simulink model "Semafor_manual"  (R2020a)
settings: Solver=VariableStepAuto  StartTime=0.0  StopTime=inf  RelTol=1e-3

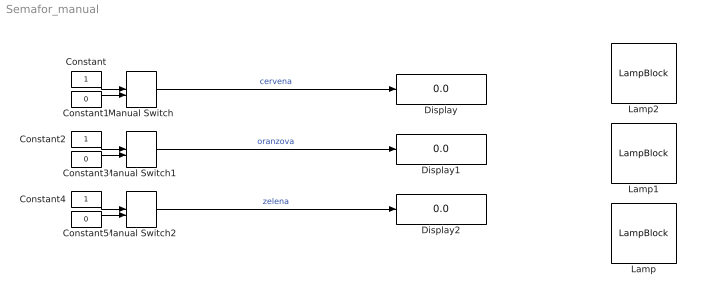
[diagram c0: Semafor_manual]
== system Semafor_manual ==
  Constant : Constant
  Constant1 : Constant  Value=0
  Constant2 : Constant
  Constant3 : Constant  Value=0
  Constant4 : Constant
  Constant5 : Constant  Value=0
  Display : Display
  Display1 : Display
  Display2 : Display
  Lamp : LampBlock  LabelPosition=Hide
  Lamp1 : LampBlock  LabelPosition=Hide
  Lamp2 : LampBlock  LabelPosition=Hide
  Manual Switch : ManualSwitch  CurrentSetting=0
  Manual Switch1 : ManualSwitch  CurrentSetting=0
  Manual Switch2 : ManualSwitch  CurrentSetting=0
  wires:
  Manual Switch/1 -> Display/1  "cervena"
  Manual Switch1/1 -> Display1/1  "oranzova"
  Manual Switch2/1 -> Display2/1  "zelena"
  Constant/1 -> Manual Switch/1
  Constant1/1 -> Manual Switch/2
  Constant3/1 -> Manual Switch1/2
  Constant2/1 -> Manual Switch1/1
  Constant4/1 -> Manual Switch2/1
  Constant5/1 -> Manual Switch2/2
